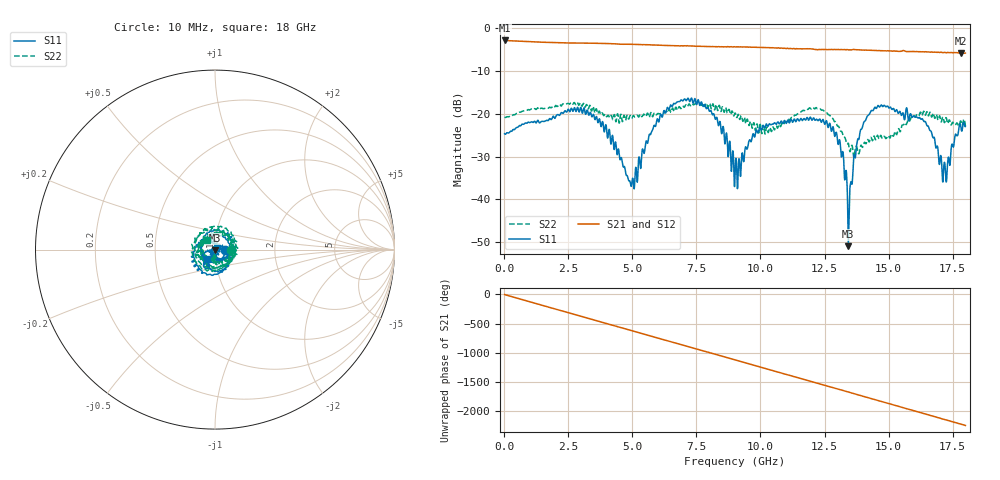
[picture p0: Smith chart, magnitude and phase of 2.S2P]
!Agilent Technologies,E5071C,MY46316741,A.11.02
!Date: Fri May 06 15:19:04 2022
!Data & Calibration Information:
!Freq	S11:SOLT2(ON)	S21:SOLT2(ON)	S12:SOLT2(ON)	S22:SOLT2(ON)
!PortZ  Port1:50+j0  Port2:50+j0
!Above PortZ is port z conversion or system Z0 setting when saving the data.
!When reading, reference impedance value at option line is always used.
# Hz S dB R 50
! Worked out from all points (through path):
!   1800 points, 10 MHz to 18 GHz, reference 50 ohm
!   highest |S21| = -2.97 dB at 10 MHz (marker M1); lowest = -6.0 dB at 17.84 GHz (marker M2)
!   group delay of S21, straight-line fit = 347 ps
!   lowest |S11| = -50.9 dB at 13.43 GHz (marker M3), VSWR 1.01, Z = 50 - j0.283 ohm
!   |S11| at or under -10 dB: start of sweep to end of sweep
!   |S22| runs from -30.2 to -17.4 dB; largest |S21 - S12| = 0.043
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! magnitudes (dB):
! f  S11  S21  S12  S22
! 10 MHz  -24.7  -3.0  -3.0  -20.8
! 3.01 GHz  -19.0  -3.6  -3.6  -18.1
! 4.03 GHz  -25.7  -3.7  -3.7  -20.5
! 5 GHz  -35.2  -3.9  -3.9  -20.8
! 6.01 GHz  -21.8  -4.0  -4.1  -20.0
! 6.96 GHz  -17.1  -4.2  -4.2  -18.2
! 7.76 GHz  -18.3  -4.3  -4.4  -17.5
! 8.48 GHz  -24.7  -4.4  -4.5  -19.1
! 9.01 GHz  -33.3  -4.5  -4.5  -19.9
! 10.04 GHz  -23.8  -4.6  -4.6  -24.4
! 12.01 GHz  -21.5  -4.9  -5.0  -18.7
! 13.02 GHz  -26.9  -5.1  -5.1  -22.9
! 13.28 GHz  -35.0  -5.1  -5.1  -25.5
! 13.43 GHz  -50.9  -5.2  -5.1  -26.9
! 13.5 GHz  -36.8  -5.2  -5.1  -28.9
! 13.72 GHz  -29.4  -5.1  -5.1  -27.7
! 13.98 GHz  -23.2  -5.2  -5.3  -27.9
! 15.01 GHz  -18.7  -5.4  -5.4  -25.2
! 16.39 GHz  -21.9  -5.7  -5.7  -19.6
! 17.19 GHz  -31.4  -5.7  -5.8  -22.1
! 17.84 GHz  -23.8  -6.0  -6.0  -22.0
! 18 GHz  -22.9  -5.9  -6.1  -22.9
